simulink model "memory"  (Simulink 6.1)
settings: Solver=ode45  StartTime=0.0  StopTime=25.0  RelTol=1e-3
undefined symbols (not defined in the file or in its folder): Bit, Location, Lower, memory_netlist, Width
libraries: xbsIndex_r3 x15, adlibrary2 x2

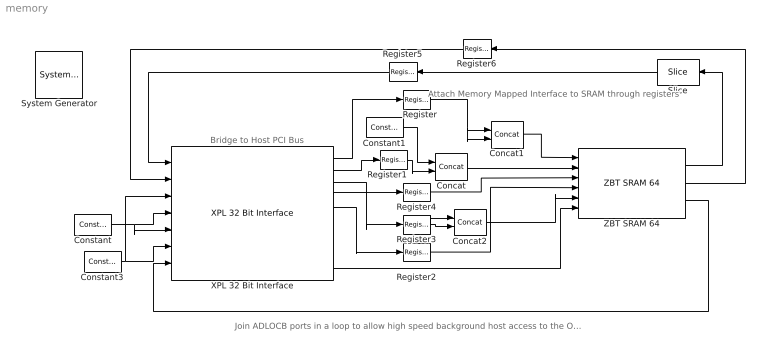
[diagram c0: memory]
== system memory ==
  note: Bridge to Host PCI Bus
  note: Attach Memory Mapped Interface to SRAM through registers
  note: Join ADLOCB ports in a loop to allow high speed background host access to the Off Chip Ram
  " System Generator" : xbsIndex_r3/ System Generator  Tag=genX  xilinxfamily=Virtex2P  part=xc2vp7  speed=-6  package=ff896  synthesis_tool=XST  directory=./memory_netlist  testbench=off  simulink_period=1  sysclk_period=7.5  incr_netlist=off  trim_vbits=Everywhere in SubSystem  dbl_ovrd=According to Block Masks  core_generation=According to Block Masks  run_coregen=off  deprecated_control=off  eval_field=0
  Concat : xbsIndex_r3/Concat  num_inputs=2  explicit_period=off  period=1  dbl_ovrd=off
  Concat1 : xbsIndex_r3/Concat  num_inputs=2  explicit_period=off  period=1  dbl_ovrd=off
  Concat2 : xbsIndex_r3/Concat  num_inputs=2  explicit_period=off  period=1  dbl_ovrd=off
  Constant : xbsIndex_r3/Constant  const=0  equ=P=C  arith_type=Boolean  n_bits=1  bin_pt=0  opselect=C  inp2=PCIN>>17  opr=+  inp1=P  carry=CIN  iostate=0  explicit_period=on  period=1  dbl_ovrd=off
  Constant1 : xbsIndex_r3/Constant  const=0  equ=P=C  arith_type=Unsigned  n_bits=4  bin_pt=0  opselect=C  inp2=PCIN>>17  opr=+  inp1=P  carry=CIN  iostate=0  explicit_period=on  period=1  dbl_ovrd=off
  Constant3 : xbsIndex_r3/Constant  const=0  equ=P=C  arith_type=Unsigned  n_bits=32  bin_pt=0  opselect=C  inp2=PCIN>>17  opr=+  inp1=P  carry=CIN  iostate=0  explicit_period=on  period=1  dbl_ovrd=off
  Register{,1..4} (5 alike) : xbsIndex_r3/Register  init=0  reg_only_valid=off  explicit_period=on  period=1  rst=off  en=off  out_en=off  dbl_ovrd=off  show_param=off
  Register5 : xbsIndex_r3/Register  Orientation=left  init=0  reg_only_valid=off  explicit_period=on  period=1  rst=off  en=off  out_en=off  dbl_ovrd=off  show_param=off
  Register6 : xbsIndex_r3/Register  Orientation=left  init=0  reg_only_valid=off  explicit_period=on  period=1  rst=off  en=off  out_en=off  dbl_ovrd=off  show_param=off
  Slice : xbsIndex_r3/Slice  Orientation=left  mode=Lower Bit Location + Width  nbits=32  bit1=0  base1=MSB of Input  bit0=0  base0=LSB of Input  boolean_output=off  explicit_period=off  period=1  dbl_ovrd=off
  XPL 32 Bit Interface : adlibrary2/ADM-XPL/XPL 32 Bit Interface  program='slave_write 0x0 0x1234;slave_read 0x0'  clock_ratio=1.5
  ZBT SRAM 64 : adlibrary2/ADM-XPL/ZBT SRAM 64
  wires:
  Constant/1 -> XPL 32 Bit Interface/5, XPL 32 Bit Interface/4
  Constant3/1 -> XPL 32 Bit Interface/3, XPL 32 Bit Interface/6
  XPL 32 Bit Interface/5 -> Register2/1
  XPL 32 Bit Interface/2 -> Register1/1
  XPL 32 Bit Interface/1 -> Register/1
  XPL 32 Bit Interface/10 -> ZBT SRAM 64/6
  ZBT SRAM 64/3 -> XPL 32 Bit Interface/7
  ZBT SRAM 64/2 -> Register6/1
  ZBT SRAM 64/1 -> Slice/1
  Register/1 -> Concat1/2, Concat1/1
  Register2/1 -> ZBT SRAM 64/4
  Register4/1 -> ZBT SRAM 64/3
  Concat/1 -> ZBT SRAM 64/2
  Constant1/1 -> Concat/1
  Register1/1 -> Concat/2
  Register5/1 -> XPL 32 Bit Interface/1
  Register6/1 -> XPL 32 Bit Interface/2
  Concat1/1 -> ZBT SRAM 64/1
  Register3/1 -> Concat2/1, Concat2/2
  Concat2/1 -> ZBT SRAM 64/5
  Slice/1 -> Register5/1
  XPL 32 Bit Interface/4 -> Register4/1
  XPL 32 Bit Interface/3 -> Register3/1
